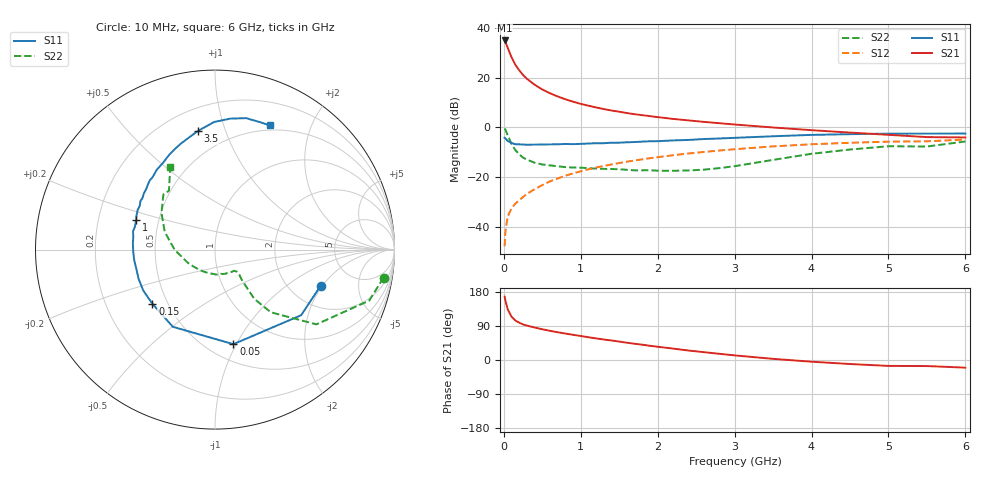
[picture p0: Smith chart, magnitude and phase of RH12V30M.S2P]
! SIEMENS Small Signal Semiconductors
! BFR106
! Si NPN RF Bipolar Junction Transistor in SOT23
! VCE = 12 V  IC = 30 mA
! Common Emitter S-Parameters:  August  1996
# GHz  S  MA  R  50
!  f  S11  S21  S12  S22
! GHz  MAG  ANG  MAG  ANG  MAG  ANG  MAG  ANG
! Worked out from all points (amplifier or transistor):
!   36 points, 10 MHz to 6 GHz, reference 50 ohm
!   highest |S21| = 34.9 dB at 10 MHz (marker M1)
!   |S21| within 3 dB of that: start of sweep to 51.16 MHz
!   unconditionally stable (mu >= 1): 341.8 MHz to 2.179 GHz
!   at 250 MHz: K = 0.93, MSG = 24.4 dB, |S12| = -27.8 dB
!   at 1.4 GHz: K = 1.07, MAG = 9.2 dB, |S12| = -14.8 dB
!   at 6 GHz: K = 0.98, MSG = 0.4 dB, |S12| = -4.8 dB
!   S11 on the Smith chart (normalised r, x): 10 MHz: 2.91, -1.92; 50 MHz: 0.66, -0.97; 150 MHz: 0.41, -0.32; 1 GHz: 0.37, +0.16; 3.5 GHz: 0.34, +0.80; 6 GHz: 0.44, +1.44
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0.01  0.6218 -19.0  55.32 167.3  0.0042 81.9  0.9524 -9.4
0.02  0.6032 -37.3  52.15 157.3  0.0081 74.0  0.9048 -18.3
0.05  0.5367 -79.0  39.57 133.7  0.0165 61.2  0.702 -36.4
0.1  0.4901 -118.6  25.43 114.4  0.024 57.2  0.4679 -48.3
0.15  0.4613 -139.1  18.02 104.1  0.0299 57.1  0.3515 -51.4
0.2  0.4601 -150.3  13.96 98.5  0.0349 60.6  0.2909 -50.4
0.25  0.4559 -158.8  11.24 93.8  0.0406 61.8  0.2492 -49.3
0.3  0.4518 -164.3  9.447 90.8  0.0467 64.4  0.2272 -48.6
0.4  0.454 -173.0  7.179 85.7  0.0582 66.5  0.1969 -46.1
0.5  0.456 -179.2  5.765 81.1  0.0702 68.1  0.1815 -44.7
0.6  0.459 175.5  4.843 77.0  0.0834 68.1  0.1739 -45.1
0.7  0.4606 171.2  4.179 73.2  0.0953 68.4  0.1673 -46.4
0.8  0.4677 167.5  3.674 69.8  0.1081 67.8  0.1609 -47.4
1  0.4696 159.6  2.971 63.3  0.1328 66.7  0.1566 -51.3
1.1  0.4778 156.0  2.728 60.0  0.1454 65.8  0.1533 -54.7
1.6  0.5054 141.5  1.944 45.6  0.2065 60.6  0.1423 -72.4
2.2  0.5504 126.1  1.484 30.1  0.2781 53.2  0.1359 -102.8
2.8  0.6019 112.1  1.219 16.4  0.3453 44.9  0.1535 -142.8
3.5  0.667 98.4  1 3.0  0.4185 35.0  0.2246 -179.6
4.5  0.7345 83.4  0.791 -10.6  0.494 20.0  0.3618 145.5
5.5  0.7532 70.3  0.642 -16.0  0.529 9.3  0.4159 128.1
6  0.7561 66.3  0.631 -20.2  0.5736 2.0  0.5245 118.4
